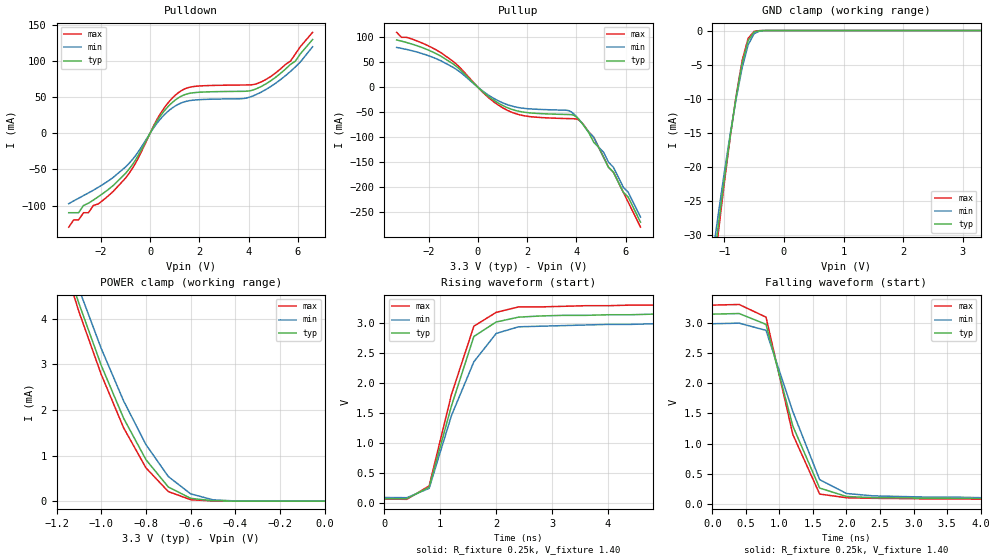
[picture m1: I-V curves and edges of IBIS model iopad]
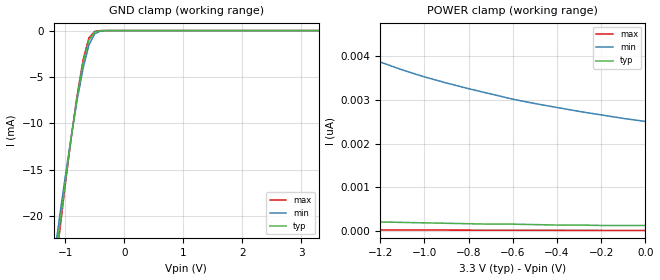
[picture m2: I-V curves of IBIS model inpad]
| IBIS file 70v3389bf.ibs created by s2ibis2 version 1.1
| North Carolina State University Electronics Research Laboratory  1995
[IBIS ver]   2.1
[File name]   70v3389bf.ibs
[File Rev]   1.0
[Date]   9/16/99 mff
[Source]   Integrated Device Technology, Inc.
[Notes]   1.Temperatures: typ=25C, min=70C, max=0C 2.RRmp rates based on
   50 ohm load.
[Disclaimer] Integrated Device Technology, Inc. ("IDT") hereby grants the
   user of this IBIS model a non-exclusive, nontransferable
   license to use this IBIS model under the following terms. The
   user is granted this license only to use the IBIS model and is
   not granted rights to sell, copy (except as needed to run the
   IBIS model), rent, lease or sub-license the IBIS model in
   whole or in part, or in modified form to anyone. The User may
   modify the IBIS model to suit its specific applications, but
   rights to derivative works and such modifications shall belong
   to IDT. This IBIS model is provided on an AS IS" basis and IDT
   makes absolutely no warranty with respect to the information
   contained herein. IDT DISCLAIMS AND CUSTOMER WAIVES ALL
   WARRANTIES, EXPRESS AND IMPLIED, INCLUDING WARRANTIES OF
   MERCHANTABILITY AND FITNESS FOR A PARTICULAR PURPOSE. THE
   ENTIRE RISK AS TO QUALITY AND PERFORMANCE IS WITH THE USER
   ACCORDINGLY, IN NO EVENT SHALL IDT BE LIABLE FOR ANY DIRECT OR
   INDIRECT DAMAGES, WHETHER IN CONTRACT OR TORT, INCLUDING A
[Copyright]   Copyright 1998, Integrated Device Technology, Inc. all rights
   reserved
|   Component test
[Component]   70v3389bf208
[Manufacturer]   Integrated Device Technology
[Package]
| variable   typ   min   max
R_pkg   100.00m   50.00m   0.30
L_pkg   4.00nH   3.20nH   5.50nH
C_pkg   0.64pF   0.50pF   0.70pF
[Pin]  signal_name   model_name   R_pin   L_pin   C_pin
A1   io9l   iopad
C2   io9r   iopad
C1   vddql   POWER
D2   vss   GND
D3   io10l   iopad
E4   io10r   iopad
E3   vddqr   POWER
F4   vss   GND
E1   io11l   iopad
F2   io11r   iopad
F1   vddql   POWER
G2   vss   GND
G3   io12l   iopad
H4   io12r   iopad
H3   vddqr   POWER
J4   vss   GND
H1   vdd   POWER
J2   vdd   POWER
J3   vss   GND
K4   vss   GND
J1   vddql   POWER
K2   vss   GND
K3   io13r   iopad
L4   io13l   iopad
K1   io14r   iopad
L2   io14l   iopad
L3   vddqr   POWER
M4   vss   GND
M3   io15r   iopad
N4   io15l   iopad
M1   vddql   POWER
N2   vss   GND
P1   io16r   iopad
P2   io16l   iopad
P3   vddqr   POWER
R1   vss   GND
R3   io17r   iopad
T2   io17l   iopad
U1   vss   GND
T3   vddql   POWER
U3   vdd   POWER
T4   vss   GND
U5   a15r   inpad
T6   a14r   inpad
R6   a13r   inpad
P7   a12r   inpad
U6   a11r   inpad
T7   a10r   inpad
R7   a9r   inpad
P8   a8r   inpad
U7   a7r   inpad
T8   be3r#   inpad
U8   be0r#   inpad
T9   ce1r   inpad
R9   ce0r   inpad
P10   vdd   POWER
U9   vdd   POWER
T10   vss   GND
R10   vss   GND
P11   clkr   inpad
U10   oer#   inpad
T11   rwr#   inpad
R11   adsr#   inpad
P12   cntenr#   inpad
U11   cntrstr#   inpad
T12   a6r   inpad
R12   a5r   inpad
P13   a4r   inpad
U12   a3r   inpad
T13   a2r   inpad
R13   a1r   inpad
U13   a0r   inpad
U14   vdd   POWER
T14   vss   GND
R14   vss   GND
U15   vdd   POWER
R15   vddql   POWER
T16   vss   GND
U17   io0l   iopad
R16   io0r   iopad
R17   vddqr   POWER
P16   vss   GND
P15   io1l   iopad
N14   io1r   iopad
N15   vddql   POWER
M14   vss   GND
N17   io2l   iopad
M16   io2r   iopad
M17   vddqr   POWER
L16   vss   GND
L15   io3l   iopad
K14   io3r   iopad
L17   io4l   iopad
K16   io4r   iopad
K15   vddql   POWER
J14   vss   GND
K17   vss   GND
J16   vss   GND
J15   vdd   POWER
H14   vdd   POWER
J17   vddqr   POWER
H16   vss   GND
H17   io5r   iopad
G16   io5l   iopad
G15   vddql   POWER
F14   vss   GND
F15   io6r   iopad
E14   io6l   iopad
F17   vddqr   POWER
E16   vss   GND
D17   io7r   iopad
D16   io7l   iopad
D15   vddql   POWER
C17   vss   GND
C15   io8r   iopad
B16   io8l   iopad
A17   vss   GND
B15   vddqr   POWER
A15   vdd   POWER
B14   vss   GND
C14   vdd   POWER
D13   vdd   POWER
A14   a0l   inpad
B13   a1l   inpad
C13   a2l   inpad
D12   a3l   inpad
A13   a4l   inpad
B12   a5l   inpad
C12   a6l   inpad
D11   cntrstl#   inpad
A12   cntenl#   inpad
B11   adsl#   inpad
C11   rwl#   inpad
D10   oel#   inpad
A11   clkl   inpad
B10   vss   GND
C10   vss   GND
D9   vdd   POWER
A10   vdd   POWER
B9   ce0l   inpad
C9   ce1l   inpad
D8   be0l#   inpad
C8   be3l#   inpad
D7   a7l   inpad
A8   a8l   inpad
B7   a9l   inpad
C7   a10l   inpad
D6   a11l   inpad
A7   a12l   inpad
B6   a13l   inpad
C6   a14l   inpad
D5   a15l   inpad
B4   vss   GND
C4   vdd   POWER
A3   vss   GND
C3   vddqr   POWER
B2   vss   GND
| in   in   dummy_model
| oe   oe   dummy_model
[Pin Mapping]  pulldown_ref   pullup_ref   gnd_clamp_ref   power_clamp_ref
A1   vss   vddql
C2   vss   vddqr
C1   NC   vddql
D2   vss   NC
D3   vss   vddql
E4   vss   vddqr
E3   NC   vddqr
F4   vss   NC
E1   vss   vddql
F2   vss   vddqr
F1   NC   vddql
G2   vss   NC
G3   vss   vddql
H4   vss   vddqr
H3   NC   vddqr
J4   vss   NC
H1   NC   vdd
J2   NC   vdd
J3   vss   NC
K4   vss   NC
J1   NC   vddql
K2   vss   NC
K3   vss   vddqr
L4   vss   vddql
K1   vss   vddqr
L2   vss   vddql
L3   NC   vddqr
M4   vss   NC
M3   vss   vddqr
N4   vss   vddql
M1   NC   vddql
N2   vss   NC
P1   vss   vddqr
P2   vss   vddql
P3   NC   vddqr
R1   vss   NC
R3   vss   vddqr
T2   vss   vddql
U1   vss   NC
T3   NC   vddql
U3   NC   vdd
T4   vss   NC
U5   vss   vdd
T6   vss   vdd
R6   vss   vdd
P7   vss   vdd
U6   vss   vdd
T7   vss   vdd
R7   vss   vdd
P8   vss   vdd
U7   vss   vdd
T8   vss   vdd
U8   vss   vdd
T9   vss   vdd
R9   vss   vdd
P10   NC   vdd
U9   NC   vdd
T10   vss   NC
R10   vss   NC
P11   vss   vdd
U10   vss   vdd
T11   vss   vdd
R11   vss   vdd
P12   vss   vdd
U11   vss   vdd
T12   vss   vdd
R12   vss   vdd
P13   vss   vdd
U12   vss   vdd
T13   vss   vdd
R13   vss   vdd
U13   vss   vdd
U14   NC   vdd
T14   vss   NC
R14   vss   NC
U15   NC   vdd
R15   NC   vddql
T16   vss   NC
U17   vss   vddql
R16   vss   vddqr
R17   NC   vddqr
P16   vss   NC
P15   vss   vddql
N14   vss   vddqr
N15   NC   vddql
M14   vss   NC
N17   vss   vddql
M16   vss   vddqr
M17   NC   vddqr
L16   vss   NC
L15   vss   vddql
K14   vss   vddqr
L17   vss   vddql
K16   vss   vddqr
K15   NC   vddql
J14   vss   NC
K17   vss   NC
J16   vss   NC
J15   NC   vdd
H14   NC   vdd
J17   NC   vddqr
H16   vss   NC
H17   vss   vddqr
G16   vss   vddql
G15   NC   vddql
F14   vss   NC
F15   vss   vddqr
E14   vss   vddql
F17   NC   vddqr
E16   vss   NC
D17   vss   vddqr
D16   vss   vddql
D15   NC   vddql
C17   vss   NC
C15   vss   vddqr
B16   vss   vddql
A17   vss   NC
B15   NC   vddqr
A15   NC   vdd
B14   vss   NC
C14   NC   vdd
D13   NC   vdd
A14   vss   vdd
B13   vss   vdd
C13   vss   vdd
D12   vss   vdd
A13   vss   vdd
B12   vss   vdd
C12   vss   vdd
D11   vss   vdd
A12   vss   vdd
B11   vss   vdd
C11   vss   vdd
D10   vss   vdd
A11   vss   vdd
B10   vss   NC
C10   vss   NC
D9   NC   vdd
A10   NC   vdd
B9   vss   vdd
C9   vss   vdd
D8   vss   vdd
C8   vss   vdd
D7   vss   vdd
A8   vss   vdd
B7   vss   vdd
C7   vss   vdd
D6   vss   vdd
A7   vss   vdd
B6   vss   vdd
C6   vss   vdd
D5   vss   vdd
B4   vss   NC
C4   NC   vdd
A3   vss   NC
C3   NC   vddqr
B2   vss   NC
| Models and submodels in the file (2): iopad (I/O), inpad (Input)
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|in   NC   NC
|oe   NC   NC
|   Model iopad
[Model]   iopad
Model_type   I/O
Polarity   Non-Inverting
Enable   Active-High
Vinl =   0.80V
Vinh =   2.00V
Vmeas =   1.50V
C_comp   1.00pF   NA   NA
[Temperature Range]   25.00   70.00   0.000
[Voltage Range]   3.30V   3.15V   3.45V
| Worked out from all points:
|   slope of the pulldown table from 0 to 0.495 V, typ, clamps not added: 18 ohm
|   slope of the pullup table from 0 to 0.495 V, typ, clamps not added: 23.7 ohm
|   GND clamp passes 1 mA (typ) near -0.56 V on its own axis
|   POWER clamp passes 1 mA (typ) near -0.81 V on its own axis
|   rising waveform, R_fixture 0.25k, V_fixture 1.40: 20-80 % time 593ps typ, 711ps min, 586ps max; typ from 0.082 V to 3.15 V
|   falling waveform, R_fixture 0.25k, V_fixture 1.40: 20-80 % time 526ps typ, 563ps min, 483ps max; typ from 3.15 V to 0.082 V
[Pulldown]
| voltage   I(typ)   I(min)   I(max)
-3.3V     -110mA     -97.5mA    -130mA
-3.1V     -110mA     -93.6mA    -120mA
-2.9V     -110mA     -90mA      -120mA
-1V       -55.69mA   -46.78mA   -62.24mA
-600mV    -37.63mA   -31.5mA    -42.12mA
400mV     22.98mA    18.97mA    26.02mA
1.1V      48.05mA    39.4mA     54.97mA
1.8V      56.39mA    46.16mA    65mA
3.8V      58.27mA    48.27mA    67mA
4.5V      64.64mA    56.89mA    71.01mA
5.7V      95.54mA    85.76mA    100mA
6.6V      130mA      120mA      140mA
[Pullup]
| voltage   I(typ)   I(min)   I(max)
-3.3V     94.72mA    79.74mA    110mA
-1.5V     62.22mA    52.99mA    69.19mA
-800mV    38.7mA     33.19mA    42.88mA
400mV     -17.28mA   -14.82mA   -19.29mA
1.2V      -40.94mA   -34.88mA   -46.19mA
2V        -50.67mA   -42.77mA   -58.01mA
3.7V      -54.58mA   -47.04mA   -62.73mA
4.1V      -64.62mA   -64.23mA   -65.64mA
4.7V      -110mA     -100mA     -100mA
4.9V      -120mA     -120mA     -120mA
6.1V      -220mA     -210mA     -230mA
6.6V      -270mA     -260mA     -280mA
[GND_clamp]
| voltage   I(typ)   I(min)   I(max)
-3.3V     -210mA     -190mA     -220mA
-1.2V     -35.67mA   -33.21mA   -37.24mA
-1.1V     -28.54mA   -26.85mA   -29.61mA
-1V       -21.76mA   -20.81mA   -22.35mA
-900mV    -15.43mA   -15.14mA   -15.59mA
-800mV    -9.68mA    -9.95mA    -9.48mA
-700mV    -4.8mA     -5.44mA    -4.39mA
-600mV    -1.48mA    -2.1mA     -1.15mA
-500mV    -210uA     -460uA     -120uA
-400mV    -17.97uA   -58.09uA   -7.86uA
-300mV    -1.11uA    -5.62uA    -350nA
3.3V      140pA      13.86nA    17.08pA
[POWER_clamp]
| voltage   I(typ)   I(min)   I(max)
-3.3V     54.48mA    50.56mA    57.22mA
-1.2V     5.85mA     6.1mA      5.73mA
-1.1V     4.34mA     4.66mA     4.16mA
-1V       2.98mA     3.35mA     2.78mA
-900mV    1.82mA     2.2mA      1.61mA
-800mV    910uA      1.24mA     730uA
-700mV    310uA      540uA      210uA
-600mV    61.42uA    160uA      31.29uA
-500mV    7.54uA     28.27uA    3.01uA
-400mV    730nA      3.93uA     220nA
0V        140pA      2.83nA     18.39pA
[Ramp]
| variable   typ   min   max
dV/dt_r   1.24/1.42n   1.10/1.61n   1.37/1.50n
dV/dt_f   1.37/1.27n   1.20/1.54n   1.50/1.16n
R_load = 50.00
[Rising Waveform]
R_fixture = 0.25k
V_fixture = 1.40
| time   V(typ)   V(min)   V(max)
0s        81.93mV    98.35mV    72.87mV
400ps     77.57mV    94.69mV    67.68mV
800ps     270mV      250mV      290mV
1.2ns     1.62V      1.46V      1.81V
1.6ns     2.77V      2.35V      2.94V
2ns       3.01V      2.82V      3.17V
2.4ns     3.09V      2.93V      3.26V
3.2ns     3.12V      2.95V      3.27V
6.8ns     3.15V      2.99V      3.3V
20ns      3.15V      2.99V      3.3V
[Falling Waveform]
R_fixture = 0.25k
V_fixture = 1.40
| time   V(typ)   V(min)   V(max)
0s        3.15V      2.99V      3.3V
400ps     3.16V      3V         3.31V
800ps     2.98V      2.88V      3.1V
1.2ns     1.29V      1.53V      1.15V
1.6ns     260mV      400mV      160mV
2ns       120mV      170mV      99.44mV
2.4ns     100mV      130mV      89.42mV
3.2ns     92.69mV    110mV      80.83mV
20ns      81.91mV    98.38mV    72.84mV
|   Model inpad
[Model]   inpad
Model_type   Input
Vinl =   0.80V
Vinh =   2.00V
C_comp   1.00pF   NA   NA
[Temperature Range]   25.00   70.00   0.000
[Voltage Range]   3.30V   3.15V   3.45V
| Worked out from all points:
|   GND clamp passes 1 mA (typ) near -0.59 V on its own axis
[GND_clamp]
| voltage   I(typ)   I(min)   I(max)
-3.3V     -150mA     -140mA     -160mA
-1.2V     -26.48mA   -24.89mA   -27.46mA
-1.1V     -21.24mA   -20.19mA   -21.89mA
-1V       -16.24mA   -15.68mA   -16.56mA
-900mV    -11.52mA   -11.43mA   -11.55mA
-800mV    -7.21mA    -7.51mA    -6.99mA
-700mV    -3.54mA    -4.1mA     -3.18mA
-600mV    -1.06mA    -1.57mA    -790uA
-500mV    -150uA     -340uA     -82.26uA
-400mV    -12.54uA   -43.03uA   -5.21uA
-300mV    -780nA     -4.21uA    -230nA
3.3V      130pA      2.62nA     15.18pA
[POWER_clamp]
| voltage   I(typ)   I(min)   I(max)
-3.3V     880pA      14.8nA     130pA
-2.9V     650pA      11.11nA    94.51pA
-2.6V     520pA      8.99nA     74.99pA
-2.1V     360pA      6.42nA     51.44pA
-1.6V     260pA      4.75nA     36.18pA
-1.5V     250pA      4.5nA      33.87pA
-1.3V     220pA      4.06nA     29.86pA
-1.1V     200pA      3.69nA     26.53pA
-1V       190pA      3.53nA     25.09pA
-800mV    170pA      3.26nA     22.58pA
-500mV    150pA      2.92nA     19.58pA
0V        130pA      2.51nA     16.01pA
